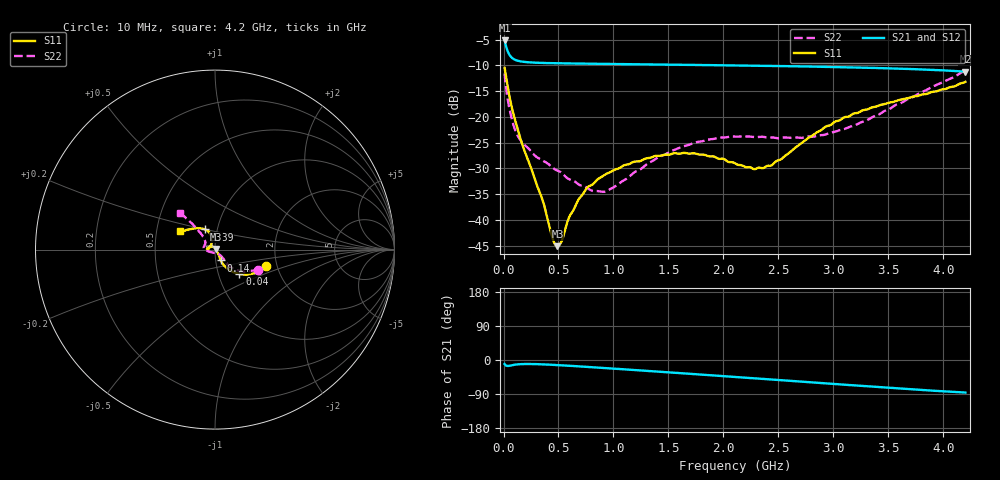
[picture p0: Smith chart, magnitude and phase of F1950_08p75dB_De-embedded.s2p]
! Integrated Device Technology
! Corporate Headquarters
! 6024 Silver Creek Valley Road
! San Jose, CA 95138  USA
! Phone:  1-408-284-8200
! Toll Free:  1-800-223-1366
! Webpage:  http://www.idt.com/
! Timing and RF Division
! 515 Groton Road, Suite 102
! Westford, MA 01886-6024
! Device:  F1950
! Description: 7-bit 0.25 dB Digital Step Attenuator
! Frequency:  150.0 -  4000.00 MHz
! Package:  4x4 mm Thin QFN Plastic Package: 24 pin
! Ports:  2 RF, 12 DC
!  Pin  1  = D0
!  Pin  2  = VDD
!  Pin  3  = Vmode
!  Pin  4  = GND
!  Pin  5  = RF1  =  Port 1
!  Pin  6  = GND
!  Pin  7  = GND
!  Pin  8  = GND
!  Pin  9  = GND
!  Pin 10  = GND
!  Pin 11  = GND
!  Pin 12  = GND
!  Pin 13  = GND
!  Pin 14  = RF2  =  Port 2
!  Pin 15  = GND
!  Pin 16  = LE
!  Pin 17  = CLK
!  Pin 18  = DATE
!  Pin 19  = D6
!  Pin 20  = D5
!  Pin 21  = D4
!  Pin 22  = D3
!  Pin 23  = D2
!  Pin 24  = D1
! State:  35
! Atten State:  8.75 dB
! Voltage:  +5.00 Volts
! Current:  Not Measured mA
! Data:  The device was measured on a the F195X evaluation board which has
!  individual transmission lines to the RF pins.  Data was collected
!  using a calibrated network analyzer.  The evaluation board was
!  de-embedded using a TRL calibration technique.
!  The reference plane is the edge of the package pin.
! Misc:  Board 2019
!  Action Tracker AT0250
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# GHz S dB R 50
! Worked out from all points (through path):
!   420 points, 10 MHz to 4.2 GHz, reference 50 ohm
!   highest |S21| = -5.14 dB at 10 MHz (marker M1); lowest = -11.2 dB at 4.2 GHz (marker M2)
!   group delay of S21, straight-line fit = 53.9 ps
!   lowest |S11| = -45.1 dB at 490 MHz (marker M3), VSWR 1.01, Z = 50.4 + j0.383 ohm
!   |S11| at or under -10 dB: start of sweep to end of sweep
!   |S22| runs from -34.6 to -11.0 dB; largest |S21 - S12| = 0.00044
!   S11 on the Smith chart (normalised r, x): 10 MHz: 1.75, -0.35; 40 MHz: 1.26, -0.36; 140 MHz: 1.06, -0.13; 3.39 GHz: 0.87, +0.20; 4.2 GHz: 0.66, +0.14
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0.01  -10.46 -17.9  -5.14 -10.7  -5.14 -10.7  -11.58 -25.4
0.04  -14.32 -45.1  -7.34 -15.7  -7.34 -15.7  -16.79 -46.5
0.09  -19.43 -59.8  -8.73 -13.1  -8.73 -13.1  -21.56 -48.4
0.14  -23.24 -61.7  -9.14 -11.2  -9.14 -11.2  -24.07 -47.2
0.36  -36.53 -38.0  -9.52 -11.5  -9.52 -11.5  -28.52 -48.7
0.45  -43.84 1.8  -9.56 -12.8  -9.56 -12.8  -29.93 -50.8
0.49  -45.13 43.3  -9.58 -13.4  -9.58 -13.4  -30.44 -53.9
0.52  -44.49 69.0  -9.59 -13.9  -9.59 -13.9  -30.73 -54.7
0.6  -39.35 104.9  -9.61 -15.3  -9.61 -15.3  -32.14 -61.1
0.71  -35.33 121.5  -9.64 -17.2  -9.64 -17.3  -33.38 -73.4
0.77  -33.58 126.6  -9.66 -18.4  -9.66 -18.4  -33.92 -81.6
0.93  -31.13 140.1  -9.70 -21.4  -9.70 -21.4  -34.47 -112.3
1.41  -27.57 168.7  -9.82 -30.8  -9.82 -30.8  -27.82 -166.9
1.74  -27.09 178.8  -9.90 -37.3  -9.90 -37.4  -25.00 -179.8
2.11  -29.10 171.4  -10.01 -44.9  -10.00 -44.9  -23.86 169.7
2.28  -30.16 152.5  -10.05 -48.3  -10.05 -48.3  -23.92 165.2
2.43  -29.49 131.8  -10.10 -51.3  -10.10 -51.3  -23.99 160.8
2.81  -23.61 105.5  -10.22 -59.1  -10.22 -59.2  -23.85 146.0
3.1  -20.06 108.4  -10.34 -65.2  -10.34 -65.2  -22.35 137.8
3.39  -17.99 117.0  -10.49 -71.1  -10.49 -71.1  -19.74 132.7
3.51  -17.21 121.5  -10.56 -73.4  -10.56 -73.5  -18.47 131.4
4.2  -13.19 152.3  -11.20 -85.9  -11.20 -85.9  -11.00 133.2
